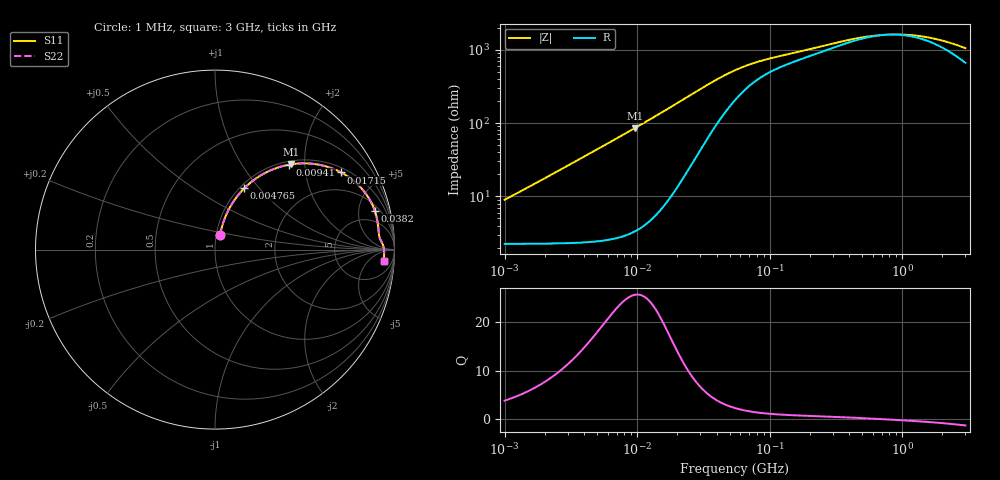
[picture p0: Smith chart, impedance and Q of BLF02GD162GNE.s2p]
! BLF02GD162GNE
# Hz S RI R 50
!Freq.(Hz) S11(Real) S11(Imag) S21(Real) S21(Imag) S12(Real) S12(Imag) S22(Real) S22(Imag)
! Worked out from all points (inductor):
!   401 points, 1 MHz to 3 GHz, reference 50 ohm
!   read as one part in series: L = 1.39 uH near 1.041 MHz
!   highest Q = 25.7 at 9.6 MHz (marker M1), where L = 1.41 uH
!   self-resonance near 787.3 MHz
!   S11 on the Smith chart (normalised r, x): 1 MHz: 1.04, +0.17; 4.765 MHz: 1.05, +0.84; 9.41 MHz: 1.07, +1.67; 17.15 MHz: 1.18, +3.15; 38.2 MHz: 2.72, +7.33; 3 GHz: 14, -16
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1000000  0.0291 0.0828  0.9709 -0.0828  0.9709 -0.0828  0.0291 0.0828
1974946  0.0492 0.1603  0.9508 -0.1603  0.9508 -0.1603  0.0492 0.1603
2831560  0.0764 0.2233  0.9236 -0.2233  0.9236 -0.2233  0.0764 0.2233
3823119  0.1172 0.2885  0.8828 -0.2885  0.8828 -0.2885  0.1172 0.2885
4764734  0.1628 0.3413  0.8372 -0.3413  0.8372 -0.3413  0.1628 0.3413
6696013  0.2674 0.4207  0.7326 -0.4207  0.7326 -0.4207  0.2674 0.4207
9410094  0.4149 0.4735  0.5851 -0.4735  0.5851 -0.4735  0.4149 0.4735
9600343  0.4246 0.4752  0.5754 -0.4752  0.5754 -0.4752  0.4246 0.4752
1.172775e7  0.5243 0.4798  0.4757 -0.4798  0.4757 -0.4798  0.5243 0.4798
1.461624e7  0.6322 0.4595  0.3678 -0.4595  0.3678 -0.4595  0.6322 0.4595
1.71545e7  0.7031 0.4297  0.2969 -0.4297  0.2969 -0.4297  0.7031 0.4297
2.509235e7  0.8269 0.329  0.1731 -0.329  0.1731 -0.329  0.8269 0.329
3.820236e7  0.89 0.2169  0.11 -0.2169  0.11 -0.2169  0.89 0.2169
5.477226e7  0.9067 0.1476  0.0933 -0.1476  0.0933 -0.1476  0.9067 0.1476
8.854986e7  0.9124 0.0931  0.0876 -0.0931  0.0876 -0.0931  0.9124 0.0931
2.094008e8  0.925 0.0481  0.075 -0.0481  0.075 -0.0481  0.925 0.0481
4.66327e8  0.9379 0.0186  0.0621 -0.0186  0.0621 -0.0186  0.9379 0.0186
8.005644e8  0.9416 -0.000602  0.0584 0.000602  0.0584 0.000602  0.9416 -0.000602
1.10276e9  0.9424 -0.0125  0.0576 0.0125  0.0576 0.0125  0.9424 -0.0125
1.519029e9  0.9424 -0.0259  0.0576 0.0259  0.0576 0.0259  0.9424 -0.0259
2.050964e9  0.9415 -0.0408  0.0585 0.0408  0.0585 0.0408  0.9415 -0.0408
3e9  0.9389 -0.0652  0.0611 0.0652  0.0611 0.0652  0.9389 -0.0652
